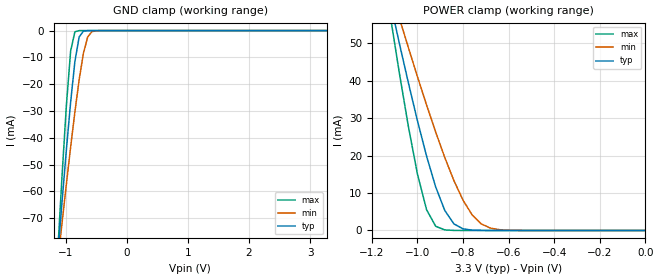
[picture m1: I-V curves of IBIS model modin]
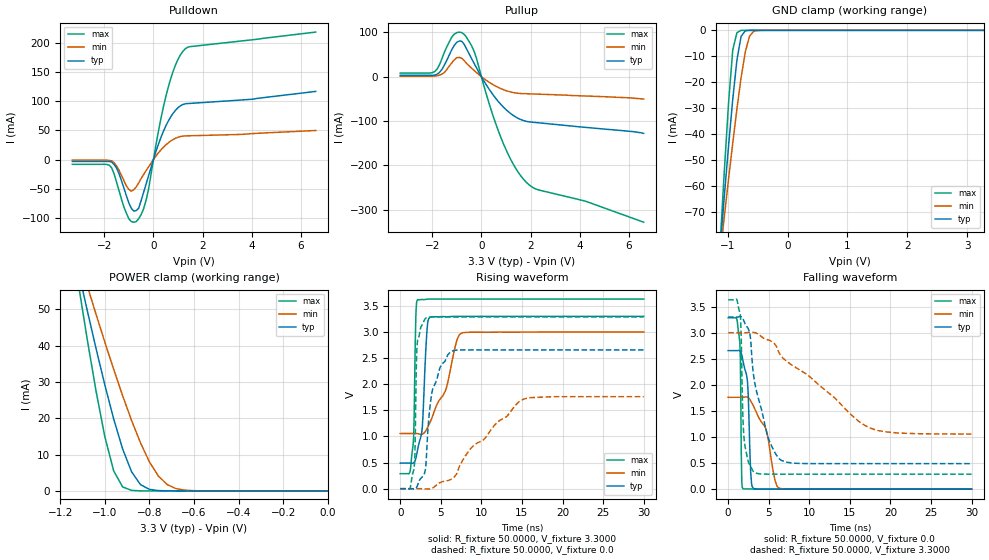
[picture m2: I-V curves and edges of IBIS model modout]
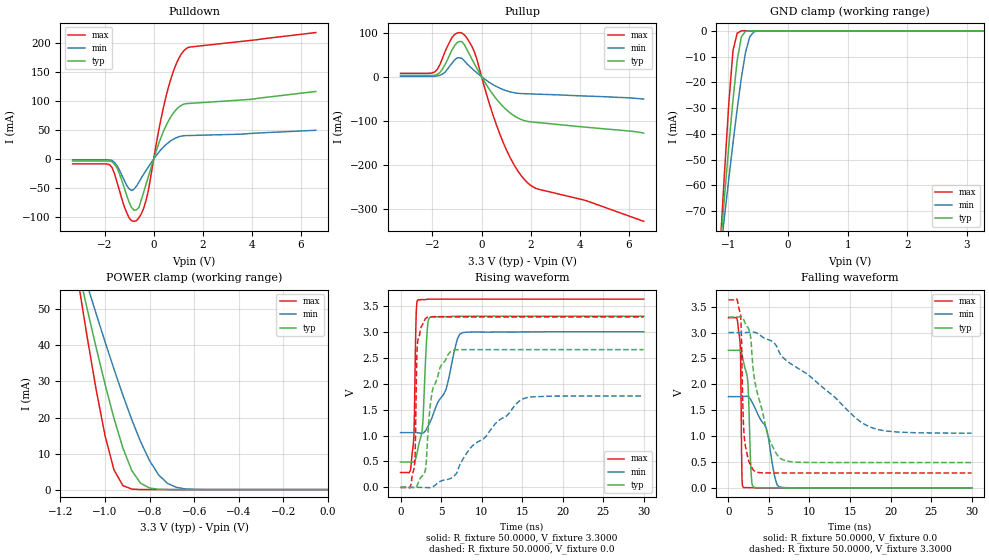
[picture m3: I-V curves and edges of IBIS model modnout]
| IBIS (I/O, Buffer, Information, Specification) Model, officially
| electronic behavioral standard for Buffer structures of digital pins.
[IBIS ver]  4.0
[File name] 54ac74_3v3_rev1.ibs
[File Rev]  1.0
[Date]   19 February 2016
[Source]   CAD & Design Services (Catania) - STMicroelectronics
[Notes]
  (Note1) This IBIS model is the model of the product with package
   (Flat14 package elements);
  (Note2) This IBIS model is extracted with nominal 3.3V power supply
   (min:3.0V, typ:3.3V, max:3.6V);
  (Note3) This model has few Warnings about the non-monotonicity
   of I-V curves, but they are not indicative of problems
   inside the model;
[Copyright] (c) 2016 STMicroelectronics
|   Component 54AC74
[Component] 54AC74
[Manufacturer] STMicroelectronics
[Package]
| variable   typ   min   max
R_pkg   0.0   0.0   0.0
L_pkg   0.0H   0.0H   0.0H
C_pkg   0.0F   0.0F   0.0F
[Pin]   signal_name   model_name   R_pin   L_pin   C_pin
1   NCD1   modin   141.0m   4.31nH   1.01pF
2   D1   modin   108.1m   3.05nH   1.04pF
3   CP1   modin   90.5m   2.36nH   0.8pF
4   NSD1   modin   79.7m   1.96nH   0.8pF
5   Q1   modout   86.2m   2.16nH   0.8pF
6   NQ1   modnout   101.7m   2.85nH   1.04pF
7   GND   GND   111.0m   3.51nH   1.01pF
8   NQ2   modnout   141.0m   4.31nH   1.01pF
9   Q2   modout   112.4m   3.25nH   1.04pF
10   NSD2   modin   90.5m   2.36nH   0.8pF
11   CP2   modin   81.9m   2.06nH   0.8pF
12   D2   modin   84.0m   2.16nH   0.8pF
13   NCD2   modin   34.7m   0.86nH   0.80pF
14   VCC   POWER   111.0m   3.51nH   1.01pF
| Models and submodels in the file (3): modin (Input), modout (I/O), modnout (I/O)
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|   Model modin
[Model]   modin
Model_type Input
Vinl   =   1.000V
Vinh   =   2.300V
C_comp   0.584pF   0.443pF   0.735pF
[Temperature Range]  25.0000   0.1250k   -55.0000
[Voltage Range]   3.3000V   3.0000V   3.6300V
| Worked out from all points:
|   GND clamp passes 1 mA (typ) near -0.74 V on its own axis
|   POWER clamp passes 1 mA (typ) near -0.82 V on its own axis
[GND_clamp]
|Voltage   I(typ)   I(min)   I(max)
-3.3V     -749mA     -568.4mA   -1.036A
-1.13V    -83.6mA    -86.25mA   -82mA
-1.06V    -63.75mA   -71.67mA   -54.05mA
-990mV    -44.61mA   -57.39mA   -28.12mA
-920mV    -26.72mA   -43.53mA   -7.666mA
-850mV    -11.52mA   -30.35mA   -438.9uA
-780mV    -2.357mA   -18.3mA    -11.16uA
-710mV    -202.6uA   -8.405mA   -269.9nA
-640mV    -13.61uA   -2.367mA   -6.525nA
-570mV    -893.7nA   -396.6uA   -166.8pA
-430mV    -3.851nA   -7.049uA   -9.072pA
3.28V     6.52pA     5.985nA    5.86pA
[POWER_clamp]
|Voltage   I(typ)   I(min)   I(max)
-3.28V    721.1mA    542.9mA    1.005A
-1.12V    61.08mA    64.91mA    57.6mA
-1.08V    50.1mA     56.8mA     42.24mA
-1.04V    39.44mA    48.83mA    27.8mA
-1V       29.27mA    41.04mA    15.03mA
-960mV    19.83mA    33.48mA    5.532mA
-920mV    11.6mA     26.24mA    1.117mA
-880mV    5.324mA    19.45mA    149.5uA
-840mV    1.752mA    13.29mA    18.09uA
-760mV    95.86uA    4.148mA    257.2nA
-680mV    4.309uA    633uA      3.657nA
0V        6.6pA      45.39pA    7.26pA
|   Model modout
[Model]   modout
Model_type I/O
Polarity   Inverting
Vinl   =   1.000V
Vinh   =   2.300V
Vmeas  =   1.65V
Cref   =   50pF
Rref   =   500
Vref   =   0
C_comp   2.925pF   2.433pF   3.856pF
[Temperature Range]  25.0000   0.1250k   -55.0000
[Voltage Range]   3.3000V   3.0000V   3.6300V
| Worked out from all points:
|   slope of the pulldown table from 0 to 0.495 V, typ, clamps not added: 8.73 ohm
|   slope of the pullup table from 0 to 0.495 V, typ, clamps not added: 11.6 ohm
|   GND clamp passes 1 mA (typ) near -0.74 V on its own axis
|   POWER clamp passes 1 mA (typ) near -0.82 V on its own axis
|   rising waveform, R_fixture 50.0000, V_fixture 3.3000: 20-80 % time 561ps typ, 2.5ns min, 237ps max; typ from 0.489 V to 3.3 V
|   rising waveform, R_fixture 50.0000, V_fixture 0.0: 20-80 % time 1.37ns typ, 6.16ns min, 232ps max; typ from 0 V to 2.66 V
|   falling waveform, R_fixture 50.0000, V_fixture 0.0: 20-80 % time 388ps typ, 1.88ns min, 142ps max; typ from 2.66 V to 0 V
|   falling waveform, R_fixture 50.0000, V_fixture 3.3000: 20-80 % time 1.97ns typ, 8.74ns min, 373ps max; typ from 3.3 V to 0.489 V
[Pulldown]
|Voltage   I(typ)   I(min)   I(max)
-3.3V     -3.244mA   -1.112mA   -8.194mA
-1.8V     -3.442mA   -1.573mA   -9.598mA
-1.5V     -14.63mA   -10.98mA   -38.85mA
-1V       -74.42mA   -51.24mA   -101.3mA
-700mV    -87.34mA   -46.76mA   -106.2mA
-600mV    -83.32mA   -39.9mA    -101.1mA
-300mV    -42.06mA   -19.04mA   -69.66mA
200mV     25.93mA    11.34mA    48mA
600mV     65.52mA    28.45mA    123.5mA
900mV     84.46mA    36.38mA    162.1mA
1.2V      94.2mA     40.13mA    185.3mA
6.6V      116.5mA    49.65mA    218mA
[Pullup]
|Voltage   I(typ)   I(min)   I(max)
-3.3V     3.024mA    1.002mA    7.894mA
-1.9V     3.315mA    1.332mA    11.19mA
-1.6V     16.6mA     5.784mA    40.99mA
-1.2V     61.13mA    31.13mA    89.43mA
-800mV    79.69mA    41.46mA    99.18mA
-300mV    30.29mA    14.12mA    57.56mA
600mV     -50.15mA   -22mA      -108.5mA
1.2V      -83.63mA   -34.73mA   -187.4mA
1.8V      -100.4mA   -38.51mA   -236.6mA
2.3V      -104mA     -39.52mA   -254.9mA
4.2V      -114.2mA   -43.69mA   -280.2mA
6.6V      -128mA     -50.57mA   -328mA
[GND_clamp]
|Voltage   I(typ)   I(min)   I(max)
-3.3V     -749mA     -568.4mA   -1.036A
-1.13V    -83.6mA    -86.23mA   -82.03mA
-1.06V    -63.76mA   -71.66mA   -54.09mA
-990mV    -44.61mA   -57.38mA   -28.11mA
-920mV    -26.71mA   -43.52mA   -7.631mA
-850mV    -11.48mA   -30.33mA   -931.7uA
-780mV    -2.332mA   -18.26mA   -10.95uA
-710mV    -199uA     -8.366mA   -266.1nA
-640mV    -13.35uA   -2.34mA    -54.4nA
-570mV    -878.5nA   -389.9uA   -23.16nA
-500mV    -57.52nA   -52.9uA    -12.08nA
3.28V     9.367pA    40.23pA    1.843pA
[POWER_clamp]
|Voltage   I(typ)   I(min)   I(max)
-3.28V    721.1mA    542.9mA    1.005A
-1.12V    61.08mA    64.9mA     57.64mA
-1.08V    50.1mA     56.79mA    42.27mA
-1.04V    39.45mA    48.82mA    27.79mA
-1V       29.26mA    41.02mA    15mA
-960mV    19.8mA     33.47mA    5.502mA
-920mV    11.56mA    26.22mA    1.109mA
-880mV    5.289mA    19.41mA    147uA
-840mV    1.737mA    13.25mA    17.76uA
-760mV    94.17uA    4.113mA    252.3nA
-680mV    4.228uA    624uA      63.07pA
0V        0A         0A         0A
[Ramp]
| variable   typ   min   max
dV/dt_r  1.5939/1.4653n   1.0570/6.1067n   1.9720/0.5278n
dV/dt_f  1.6863/2.1042n   1.1659/8.7185n   2.0055/0.4166n
R_load = 50.0000
[Rising Waveform]
R_fixture= 50.0000
V_fixture= 3.3000
V_fixture_min= 3.0000
V_fixture_max= 3.6300
|time   V(typ)   V(min)   V(max)
0s        489.4mV    1.057V     287.5mV
1.2ns     489.8mV    1.057V     317.7mV
1.59ns    489mV      1.057V     848mV
1.92ns    581.1mV    1.057V     3.277V
2.13ns    734.9mV    1.054V     3.615V
2.73ns    1.201V     1.047V     3.623V
3.27ns    2.971V     1.141V     3.627V
3.63ns    3.278V     1.252V     3.63V
7.65ns    3.3V       2.983V     3.63V
30ns      3.3V       3V         3.63V
[Rising Waveform]
R_fixture= 50.0000
V_fixture= 0.0
V_fixture_min= 0.0
V_fixture_max= 0.0
|time   V(typ)   V(min)   V(max)
0s        132.2pV    0V         79.98pV
1.68ns    -5.755mV   -46.22uV   367.5mV
1.8ns     -7.062mV   13.83uV    605.2mV
1.95ns    10.96mV    273.6uV    2.09V
2.07ns    41.2mV     485.3uV    2.741V
3.15ns    434.5mV    -3.946mV   3.266V
3.93ns    1.858V     6.745mV    3.286V
6.21ns    2.622V     173.9mV    3.287V
15.27ns   2.657V     1.717V     3.287V
30ns      2.657V     1.762V     3.287V
[Falling Waveform]
R_fixture= 50.0000
V_fixture= 0.0
V_fixture_min= 0.0
V_fixture_max= 0.0
|time   V(typ)   V(min)   V(max)
0s        2.657V     1.762V     3.287V
1.44ns    2.654V     1.761V     2.807V
1.5ns     2.642V     1.761V     2.526V
1.68ns    2.571V     1.761V     137.1mV
1.86ns    2.435V     1.763V     6.596mV
2.4ns     2.024V     1.765V     4.27mV
2.79ns    298.6mV    1.691V     4.613mV
3.12ns    13.99mV    1.593V     2.921mV
6.24ns    1.697mV    21.91mV    214.6nV
30ns      -12.16nV   1.19uV     -1.37uV
[Falling Waveform]
R_fixture= 50.0000
V_fixture= 3.3000
V_fixture_min= 3.0000
V_fixture_max= 3.6300
|time   V(typ)   V(min)   V(max)
0s        3.3V       3V         3.63V
1.5ns     3.311V     3V         3.34V
1.8ns     3.272V     3V         1.457V
1.98ns    3.211V     2.999V     939.3mV
2.7ns     2.952V     3.007V     460.1mV
3.24ns    2.073V     3.003V     322.4mV
4.98ns    961.9mV    2.859V     287.9mV
6.66ns    545.6mV    2.527V     287.5mV
17.34ns   489.4mV    1.183V     287.5mV
30ns      489.4mV    1.057V     287.5mV
|   Model modnout
[Model]   modnout
Model_type I/O
Polarity   Non-Inverting
Vinl   =   1.000V
Vinh   =   2.300V
Vmeas  =   1.65V
Cref   =   50pF
Rref   =   500
Vref   =   0
C_comp   2.925pF   2.433pF   3.856pF
[Temperature Range]  25.0000   0.1250k   -55.0000
[Voltage Range]   3.3000V   3.0000V   3.6300V
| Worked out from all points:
|   slope of the pulldown table from 0 to 0.495 V, typ, clamps not added: 8.73 ohm
|   slope of the pullup table from 0 to 0.495 V, typ, clamps not added: 11.6 ohm
|   GND clamp passes 1 mA (typ) near -0.74 V on its own axis
|   POWER clamp passes 1 mA (typ) near -0.82 V on its own axis
|   rising waveform, R_fixture 50.0000, V_fixture 3.3000: 20-80 % time 561ps typ, 2.5ns min, 237ps max; typ from 0.489 V to 3.3 V
|   rising waveform, R_fixture 50.0000, V_fixture 0.0: 20-80 % time 1.37ns typ, 6.16ns min, 232ps max; typ from 0 V to 2.66 V
|   falling waveform, R_fixture 50.0000, V_fixture 0.0: 20-80 % time 388ps typ, 1.88ns min, 142ps max; typ from 2.66 V to 0 V
|   falling waveform, R_fixture 50.0000, V_fixture 3.3000: 20-80 % time 1.97ns typ, 8.74ns min, 373ps max; typ from 3.3 V to 0.489 V
[Pulldown]
|Voltage   I(typ)   I(min)   I(max)
-3.3V     -3.244mA   -1.112mA   -8.194mA
-1.8V     -3.442mA   -1.573mA   -9.598mA
-1.5V     -14.63mA   -10.98mA   -38.85mA
-1V       -74.42mA   -51.24mA   -101.3mA
-700mV    -87.34mA   -46.76mA   -106.2mA
-600mV    -83.32mA   -39.9mA    -101.1mA
-300mV    -42.06mA   -19.04mA   -69.66mA
200mV     25.93mA    11.34mA    48mA
600mV     65.52mA    28.45mA    123.5mA
900mV     84.46mA    36.38mA    162.1mA
1.2V      94.2mA     40.13mA    185.3mA
6.6V      116.5mA    49.65mA    218mA
[Pullup]
|Voltage   I(typ)   I(min)   I(max)
-3.3V     3.024mA    1.002mA    7.894mA
-1.9V     3.315mA    1.332mA    11.19mA
-1.6V     16.6mA     5.784mA    40.99mA
-1.2V     61.13mA    31.13mA    89.43mA
-800mV    79.69mA    41.46mA    99.18mA
-300mV    30.29mA    14.12mA    57.56mA
600mV     -50.15mA   -22mA      -108.5mA
1.2V      -83.63mA   -34.73mA   -187.4mA
1.8V      -100.4mA   -38.51mA   -236.6mA
2.3V      -104mA     -39.52mA   -254.9mA
4.2V      -114.2mA   -43.69mA   -280.2mA
6.6V      -128mA     -50.57mA   -328mA
[GND_clamp]
|Voltage   I(typ)   I(min)   I(max)
-3.3V     -749mA     -568.4mA   -1.036A
-1.13V    -83.6mA    -86.23mA   -82.03mA
-1.06V    -63.76mA   -71.66mA   -54.09mA
-990mV    -44.61mA   -57.38mA   -28.11mA
-920mV    -26.71mA   -43.52mA   -7.631mA
-850mV    -11.48mA   -30.33mA   -931.7uA
-780mV    -2.332mA   -18.26mA   -10.95uA
-710mV    -199uA     -8.366mA   -266.1nA
-640mV    -13.35uA   -2.34mA    -54.4nA
-570mV    -878.5nA   -389.9uA   -23.16nA
-500mV    -57.52nA   -52.9uA    -12.08nA
3.28V     9.367pA    40.23pA    1.843pA
[POWER_clamp]
|Voltage   I(typ)   I(min)   I(max)
-3.28V    721.1mA    542.9mA    1.005A
-1.12V    61.08mA    64.9mA     57.64mA
-1.08V    50.1mA     56.79mA    42.27mA
-1.04V    39.45mA    48.82mA    27.79mA
-1V       29.26mA    41.02mA    15mA
-960mV    19.8mA     33.47mA    5.502mA
-920mV    11.56mA    26.22mA    1.109mA
-880mV    5.289mA    19.41mA    147uA
-840mV    1.737mA    13.25mA    17.76uA
-760mV    94.17uA    4.113mA    252.3nA
-680mV    4.228uA    624uA      63.07pA
0V        0A         0A         0A
[Ramp]
| variable   typ   min   max
dV/dt_r  1.5939/1.4653n   1.0570/6.1067n   1.9720/0.5278n
dV/dt_f  1.6863/2.1042n   1.1659/8.7185n   2.0055/0.4166n
R_load = 50.0000
[Rising Waveform]
R_fixture= 50.0000
V_fixture= 3.3000
V_fixture_min= 3.0000
V_fixture_max= 3.6300
|time   V(typ)   V(min)   V(max)
0s        489.4mV    1.057V     287.5mV
1.2ns     489.8mV    1.057V     317.7mV
1.59ns    489mV      1.057V     848mV
1.92ns    581.1mV    1.057V     3.277V
2.13ns    734.9mV    1.054V     3.615V
2.73ns    1.201V     1.047V     3.623V
3.27ns    2.971V     1.141V     3.627V
3.63ns    3.278V     1.252V     3.63V
7.65ns    3.3V       2.983V     3.63V
30ns      3.3V       3V         3.63V
[Rising Waveform]
R_fixture= 50.0000
V_fixture= 0.0
V_fixture_min= 0.0
V_fixture_max= 0.0
|time   V(typ)   V(min)   V(max)
0s        132.2pV    0V         79.98pV
1.68ns    -5.755mV   -46.22uV   367.5mV
1.8ns     -7.062mV   13.83uV    605.2mV
1.95ns    10.96mV    273.6uV    2.09V
2.07ns    41.2mV     485.3uV    2.741V
3.15ns    434.5mV    -3.946mV   3.266V
3.93ns    1.858V     6.745mV    3.286V
6.21ns    2.622V     173.9mV    3.287V
15.27ns   2.657V     1.717V     3.287V
30ns      2.657V     1.762V     3.287V
[Falling Waveform]
R_fixture= 50.0000
V_fixture= 0.0
V_fixture_min= 0.0
V_fixture_max= 0.0
|time   V(typ)   V(min)   V(max)
0s        2.657V     1.762V     3.287V
1.44ns    2.654V     1.761V     2.807V
1.5ns     2.642V     1.761V     2.526V
1.68ns    2.571V     1.761V     137.1mV
1.86ns    2.435V     1.763V     6.596mV
2.4ns     2.024V     1.765V     4.27mV
2.79ns    298.6mV    1.691V     4.613mV
3.12ns    13.99mV    1.593V     2.921mV
6.24ns    1.697mV    21.91mV    214.6nV
30ns      -12.16nV   1.19uV     -1.37uV
[Falling Waveform]
R_fixture= 50.0000
V_fixture= 3.3000
V_fixture_min= 3.0000
V_fixture_max= 3.6300
|time   V(typ)   V(min)   V(max)
0s        3.3V       3V         3.63V
1.5ns     3.311V     3V         3.34V
1.8ns     3.272V     3V         1.457V
1.98ns    3.211V     2.999V     939.3mV
2.7ns     2.952V     3.007V     460.1mV
3.24ns    2.073V     3.003V     322.4mV
4.98ns    961.9mV    2.859V     287.9mV
6.66ns    545.6mV    2.527V     287.5mV
17.34ns   489.4mV    1.183V     287.5mV
30ns      489.4mV    1.057V     287.5mV
